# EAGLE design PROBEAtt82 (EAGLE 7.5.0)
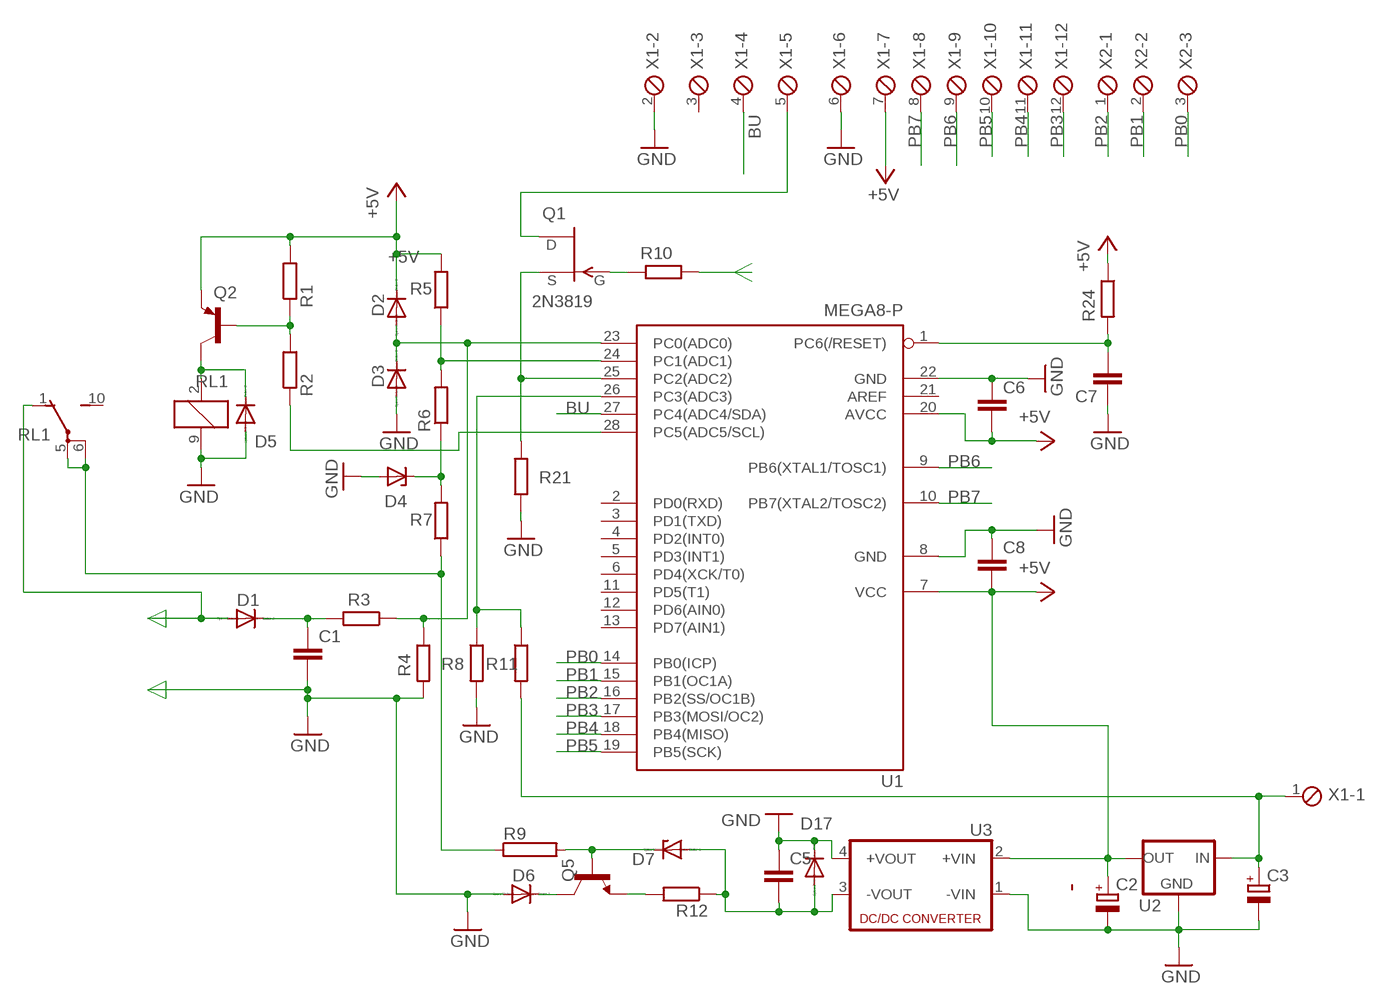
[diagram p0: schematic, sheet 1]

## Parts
C1  C-EU150-091X182  [C150-091X182]
C2  CPOL-EUE2-5  [E2-5]
C3  CPOL-EUE2-5  [E2-5]
C5  C-EUC1206  [C1206]
C6  C-EUC1206  [C1206]
C7  C-EUC1206  [C1206]
C8  C-EUC1206  [C1206]
D1  1N4004  [DO41-10]
D2  1N4004  [DO41-10]
D3  1N4004  [DO41-10]
D4  ZY  [P1Z12]
D5  1N4004  [DO41-10]
D6  1N4004  [DO41-10]
D7  DIODE-DO214AA  [DO214AA]
D17  DIODE-DO214AA  [DO214AA]
Q1  2N3819  [TO92]
Q2  BC327  [TO92]
Q5  -NPN-TO126  [TO126]
R1  R-EU_0204/7  [0204/7]
R2  R-EU_0204/7  [0204/7]
R3  R-EU_0617/22  [0617/22]
R4  R-EU_0411/12  [0411/12]
R5  R-EU_0204/7  [0204/7]
R6  R-EU_0204/7  [0204/7]
R7  R-EU_0414/15  [0414/15]
R8  R-EU_0204/7  [0204/7]
R9  RHPS932  [HPS932]
R10  R-EU_0204/7  [0204/7]
R11  R-EU_0204/7  [0204/7]
R12  R-EU_0204/7  [0204/7]
R21  R-EU_0204/7  [0204/7]
R24  R-EU_0204/7  [0204/7]
RL1  G5V1  [G5V1]
U1  MEGA8-P  [DIL28-3]
U2  78XXL  [78XXL]
U3  NME  [NME]
X1  MPT12  [12POL254]
X2  MPT3  [3POL254]

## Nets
+5V: C2.+ C6.2 C8.2 D2.C Q2.1(E) R1.2 R5.2 R24.1 U1.7(VCC) U1.20(AVCC) U2.OUT U3.2(+VIN) X1.7
BU: U1.27(PC4(ADC4/SDA)) X1.4
GND: C1.2 C2.- C3.- C5.1 C6.1 C7.1 C8.1 D3.A D4.A D5.A D6.A D17.C R4.2 R8.2 R21.2 RL1.9 U1.8(GND) U1.22(GND) U2.GND U3.1(-VIN) U3.4(+VOUT) X1.2 X1.6
N$1: R8.1 R11.1 U1.26(PC3(ADC3))
N$2: Q1.1(D) X1.5
N$3: C7.2 R24.2 U1.1(PC6(/RESET))
N$5: R5.1 R6.2 U1.24(PC1(ADC1))
N$6: D7.C Q5.3(B) R9.2
N$7: D4.C R6.1 R7.2
N$8: C1.1 D1.C R3.2
N$10: R2.1 U1.28(PC5(ADC5/SCL))
N$12: D5.C Q2.3(C) RL1.2
N$13: Q1.3(S) R21.1 U1.25(PC2(ADC2))
N$15: Q2.2(B) R1.1 R2.2
N$16: R7.1 R9.1 RL1.5(2:P) RL1.6(2:P)
N$18: C3.+ R11.2 U2.IN X1.1
N$19: D2.A D3.C R3.1 R4.1 U1.23(PC0(ADC0))
N$21: Q1.2(G) R10.2
N$28: C5.2 D7.A D17.A R12.1 U3.3(-VOUT)
N$30: Q5.1(E) R12.2
N$31: D6.C Q5.2(C)
N$32: R10.1
N$33: D1.A RL1.1(2:O)
PB0: U1.14(PB0(ICP)) X2.3
PB1: U1.15(PB1(OC1A)) X2.2
PB2: U1.16(PB2(SS/OC1B)) X2.1
PB3: U1.17(PB3(MOSI/OC2)) X1.12
PB4: U1.18(PB4(MISO)) X1.11
PB5: U1.19(PB5(SCK)) X1.10
PB6: U1.9(PB6(XTAL1/TOSC1)) X1.9
PB7: U1.10(PB7(XTAL2/TOSC2)) X1.8
Unconnected: RL1.10(2:S) U1.2(PD0(RXD)) U1.3(PD1(TXD)) U1.4(PD2(INT0)) U1.5(PD3(INT1)) U1.6(PD4(XCK/T0)) U1.11(PD5(T1)) U1.12(PD6(AIN0)) U1.13(PD7(AIN1)) U1.21(AREF) X1.3

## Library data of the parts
C1 C5-C8 = rcl:C-EU: CAPACITOR, European symbol
C2 C3 = rcl:CPOL-EU: POLARIZED CAPACITOR, European symbol
D1-D3 D5 D6 = diode:1N4004: DIODE
D4 = diode:ZY: Z DIODE
D7 D17 = diode:DIODE-: DIODE
Q1 = transistor-fet:2N3819: N-Channel Junction FET
Q2 = transistor-pnp:BC327: PNP Transistor
Q5 = transistor:*-NPN-: NPN Transistror BF959 corrected 2008.03.06
R1-R8 R10-R12 R21 R24 = rcl:R-EU_: RESISTOR, European symbol
R9 = resistor-power:R: Power Resitor; OC_FARNELL: unknown; OC_NEWARK: unknown
RL1 = relay:G5V1: RELAY 1 x switch, 0.5 A/125 V AC, 1 A/24 V DC , Omron; MPN: G5V-1-DC24; OC_FARNELL: 9949593; OC_NEWARK: 36M6377
U1 = atmel:MEGA8-P: MICROCONTROLLER 8 Kbytes FLASH, 1 kbytes SRAM, 512 bytes EEPROM, USART, 4-channel 10 bit ADC, 2-channel 8 bit ADC Pin compatible with Atmega48, ATMega88, ATMega168 Source: avr.lbr; OC_FARNELL: unknown; OC_NEWARK: unknown
U2 = v-reg:78XXL: VOLTAGE REGULATOR
U3 = dc-dc-converter:NME: DC-DC CONVERTER; MF: C & D TECHNOLOGIES, INC; MPN: NME1205D; OC_FARNELL: 1021466; OC_NEWARK: 98B8198
X1 = con-phoenix-254:MPT12: PHOENIX CONNECTOR; OC_FARNELL: unknown; OC_NEWARK: unknown
X2 = con-phoenix-254:MPT3: PHOENIX CONNECTOR; OC_FARNELL: unknown; OC_NEWARK: unknown

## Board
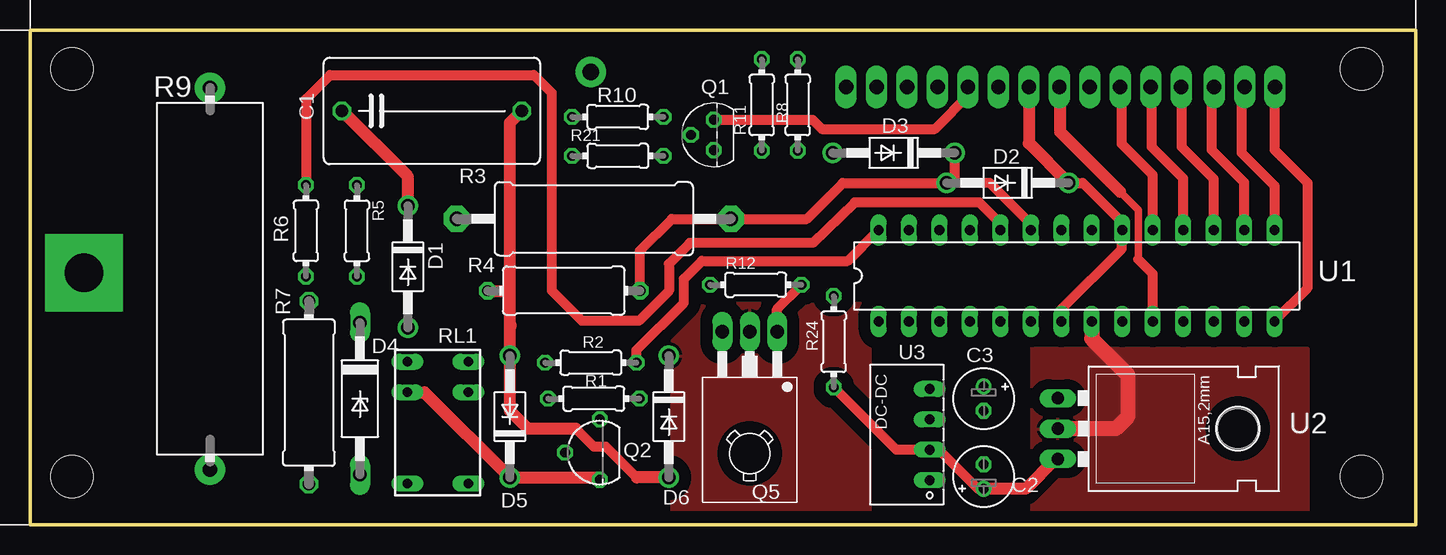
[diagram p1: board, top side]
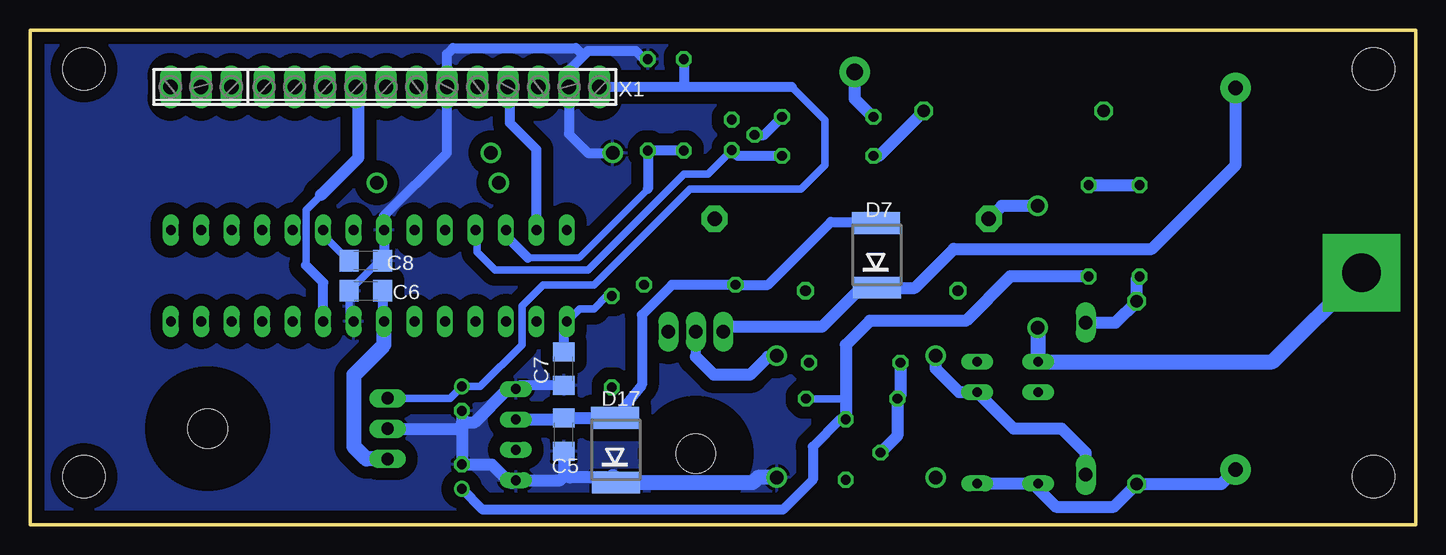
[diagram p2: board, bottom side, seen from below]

Size 115.5 x 41.25 mm. Coordinates in mm from the lower left corner, seen from the top.
Outline: 0,0 0,41.25 115.5,41.25 115.5,0 0,0
Copper layers (1*16): Top 0.035mm / dielectric 1.5mm / Bottom 0.035mm
Design rules "default": minimum track width 10mil, minimum drill 24mil, track to track 8mil, track to pad 8mil, pad to pad 8mil, via to via 8mil, smd to smd 8mil, copper to edge 40mil, drill to drill 8mil, minimum pad ring 10mil, minimum via ring 8mil, stop-mask expansion 4mil, vias tented up to drill 0mil, thermal gap 10mil
Holes 3.5 mm at 3.5,38 3.5,4 111,4 111,38

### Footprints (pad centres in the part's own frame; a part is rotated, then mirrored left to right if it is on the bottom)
C150-091X182 = drill 1.016 octagon: 1 -7.493,0; 2 7.493,0
E2-5 = drill 0.813 pad 1.27: + -1.016,0 | drill 0.813 pad 1.27 octagon: - 1.016,0
C1206 = smd 1.6 x 1.8: 1 -1.4,0; 2 1.4,0
DO41-10 = drill 1.118: A 5.08,0; C -5.08,0
P1Z12 = drill 1.118 long: A 6.35,0; C -6.35,0
DO214AA = smd 1.8 x 4: A 2.65,0; C -2.75,-0.1
TO92 = drill 0.813 octagon: 1 1.27,0; 2 0,1.905; 3 -1.27,0
TO92' = drill 0.813 octagon: 1 2.77,0; 2 0,2.905; 3 -2.27,0
TO126 = drill 1.118 long: 1 -2.286,-5.08; 2 0,-5.08; 3 2.286,-5.08 | hole 3.302: 0,5.08
0204/7 = drill 0.813 octagon: 1 -3.81,0; 2 3.81,0
0617/22 = drill 1.2 pad 2.184 octagon: 1 -11.43,0; 2 11.43,0
0411/12 = drill 0.914 octagon: 1 -6.35,0; 2 6.35,0
0414/15 = drill 1.016 octagon: 1 -7.62,0; 2 7.62,0
HPS932 = drill 1.2 pad 2.54: 1 -15.93,0; 2 15.93,0
G5V1 = drill 0.813 long: 1 -5.08,-2.54; 2 -2.54,-2.54; 5 5.08,-2.54; 6 5.08,2.54; 9 -2.54,2.54; 10 -5.08,2.54
DIL28-3 = drill 0.813 long: 1 -16.51,-3.81; 2 -13.97,-3.81; 3 -11.43,-3.81; 4 -8.89,-3.81; 5 -6.35,-3.81; 6 -3.81,-3.81; 7 -1.27,-3.81; 8 1.27,-3.81; 9 3.81,-3.81; 10 6.35,-3.81; 11 8.89,-3.81; 12 11.43,-3.81; 13 13.97,-3.81; 14 16.51,-3.81; 15 16.51,3.81; 16 13.97,3.81; 17 11.43,3.81; 18 8.89,3.81; 19 6.35,3.81; 20 3.81,3.81; 21 1.27,3.81; 22 -1.27,3.81; 23 -3.81,3.81; 24 -6.35,3.81; 25 -8.89,3.81; 26 -11.43,3.81; 27 -13.97,3.81; 28 -16.51,3.81
78XXL = drill 1.016 long: GND 0,-3.81; IN -2.54,-3.81; OUT 2.54,-3.81 | hole 3.302: 0,11.176
NME = drill 0.813 long: 1 0,3.81; 2 0,1.27; 3 0,-1.27; 4 0,-3.81
12POL254 = drill 1.2 long: 1 -13.97,0; 2 -11.43,0; 3 -8.89,0; 4 -6.35,0; 5 -3.81,0; 6 -1.27,0; 7 1.27,0; 8 3.81,0; 9 6.35,0; 10 8.89,0; 11 11.43,0; 12 13.97,0
3POL254 = drill 1.2 long: 1 -2.54,0; 2 0,0; 3 2.54,0

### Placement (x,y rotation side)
C1  33.5,34.5 0 top
C2  79.5,4 90 top
C3  79.5,10.5 270 top
C5  71,7.5 90 bottom
C6  87.5,19.5 0 bottom
C7  71,13 90 bottom
C8  87.5,22 180 bottom
D1  31.5,21.5 270 top
D2  81.5,28.5 180 top
D3  72,31 180 top
D4  27.5,10.5 270 top
D5  40,9 90 top
D6  53.25,9 270 top
D7  45,22.5 90 bottom
D17  66.75,6.25 90 bottom
Q1  57,32.5 90 top
Q2  BC327  [TO92']  47.5,6 90 top
Q5  60,11 180 top
R1  47,10.5 0 top
R2  46.75,13.5 180 top
R3  47,25.5 180 top
R4  44.5,19.5 180 top
R5  27.25,24.5 270 top
R6  23,24.5 90 top
R7  23.25,11 90 top
R8  64,35 90 top
R9  15,20.5 90 top
R10  49,34 0 top
R11  61,35 90 top
R12  60.5,20 0 top
R21  49,30.75 180 top
R24  67,15.25 90 top
RL1  34,8.5 270 top
U1  87.25,20.75 0 top
U2  89.5,8 270 top
U3  75,7.5 180 top
X1  82,36.5 180 bottom
X2  101.25,36.5 180 bottom

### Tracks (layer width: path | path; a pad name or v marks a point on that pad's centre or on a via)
+5V
  Top 0.813: C2.+ 79.48,3 79,3 75.77,6.23 U3.2 72.21,6.23 R24.1 | U1.7 85.98,17.98 91,23 91,24.5 U1.20 91,24.62 91,25.25 87.75,28.5 87.12,28.5
  Top 1.016: U2.OUT 85.46,5.46 83,3 79.52,3 C2.+ | X1.7 83.27,31.81 D2.C 87.12,28.5
  Bottom 0.61: U1.20 91.06,24.16 C8.2 | R1.2 47.5,10.5
  Bottom 0.813: C6.2 86.1,17.06 U1.7 | Q2.1 47.98,8.77 50.25,6.5 50.25,3.75 52.75,1.25 77.77,1.25 C2.+
  Bottom 1.016: R5.2 33.81,20.69 37.5,17 45.5,17 47.5,15 47.5,10.5 Q2.1
  Bottom 1.27: U2.OUT 87.46,5.46 88.5,6.5 88.5,12.5 86,15 86,16.92 U1.7
BU
  Bottom 0.813: U1.27 73.28,31.28 75.5,33.5 75.5,35.85 X1.4
GND
  Top 0.813: 50.58,3.92 48,6.5 47,6.5 45.5,8
  Top 1.016: 40,16.5 D5.A 40,9.5 41.5,8 45.5,8 | 40,16.5 40,19.5 | 40,19.5 40,33.51 C1.2 | R4.2 40,19.5 | 40.08,16.58 40,16.5 | D6.A 50.58,3.92
  Top 1.27: U1.8 88.52,15.48 91.5,12.5 91.5,9 90.5,8 U2.GND
  Bottom 0.61: C8.1 86.4,22 C6.1 88.9,17.32 U1.8
  Bottom 0.813: C7.1 74.71,11.6 U3.4 | R8.2 64.31,38.81 65,39.5 69,39.5 69.38,39.12 | 69.38,39.12 70.5,38 70.5,36.57 X1.2 70.57,32.57 69,31 D3.A | C8.1 85.98,22.12 U1.22 85.98,25.77 80.75,31 80.75,36.48 X1.6 80.73,39.23 80.75,39.25 80.25,39.75 70,39.75 69.38,39.12
  Bottom 1.016: R21.2 44.74,30.75 C1.2 | D5.A 40,13 38.04,11.04 RL1.9 33.5,8 29.5,8 27.5,6 D4.A | C5.1 71,4.42 70.79,4.21 | 70.79,4.21 70.5,3.92 67,3.92 66.9,4.02 D17.C | 70.79,4.21 71.31,3.69 U3.1 75.19,3.5 75.5,3.5 77.02,5.02 C2.- 79.5,8 | C3.- 79.5,8.5 | 79.5,8.5 79.5,8 | U2.GND 79.5,8 | U3.4 75.69,11.31 78.5,8.5 79.5,8.5
  Bottom 1.27: D6.A 54.83,3.92 55.25,3.5 66.38,3.5 66.9,4.02
  pour Bottom (isolate 1.016): 50.5,40.5 114.75,40.5 114.75,0.75 50.5,0.75
  pour Top (isolate 0.813): 106.5,14.75 106.5,1 83.5,1 83.5,14.75
N$1
  Bottom 0.6: 64,28 69.75,22.25 74,22.25
  Bottom 0.813: R11.1 R8.1 64,28 | 74,22.25 75.75,24 75.75,24.49 U1.26
N$2
  Top 0.813: Q1.1 65.23,33.77 66,33 75.44,33 78.4,35.96 | 78.5,35.69 78.4,35.96 | 78.4,35.96 X1.5
N$3
  Bottom 0.61: R24.2 67.44,19.06 68.5,18 69.68,18 U1.1
  Bottom 0.813: C7.2 71,16.68 U1.1
N$4  (via drill 1.4 pad 2.54)
  Bottom 1.016: 45.25,34 46.75,35.5 v46.75,37.75 47,37.75
N$5
  Top 0.813: U1.24 80.9,25.1 79.12,26.88 68.75,26.88 65.25,23.5 55,23.5 53.25,21.75 53.25,19.5 50.75,17 46,17 43.5,19.5 43.5,36 42,37.5 25,37.5 23,35.5 R6.2
  Bottom 1.016: R5.1 R6.2
N$6
  Bottom 1.016: R9.2 15,30 22,23 38.5,23 41.75,19.75 D7.C 46.25,19.75 49.5,16.5 57.29,16.5 Q5.3
N$7
  Bottom 1.016: R6.1 23.25,20.44 R7.2 25.02,16.85 D4.C
N$8
  Top 1.016: D1.C 31.5,29.01 C1.1
  Bottom 1.016: D1.C 34.49,26.58 R3.2
N$10
  Top 0.813: R2.1 50.56,14.56 54.5,18.5 54.5,20.5 56,22 68.18,22 U1.28
N$12
  Top 1.016: RL1.2 32.88,11.04 D5.C 47.31,3.92 Q2.3
N$13
  Bottom 0.61: U1.25 78.25,24.45 78.25,22.75 76.75,21.25 69,21.25 61,29.25 58.98,29.25 Q1.3
  Bottom 0.813: R21.1 56.52,30.75 Q1.3 57.02,31.23
N$15
  Bottom 1.016: R2.2 42.94,10.75 R1.1 43.19,7.41 Q2.2
N$16
  Bottom 1.016: RL1.6 RL1.5 31.46,2.96 30,1.5 25.13,1.5 R7.1 16.19,3.38 R9.1
N$18
  Bottom 0.61: U2.IN 80.48,10.54 C3.+ 77.98,11.52 74.5,15 74.5,18.25 72.75,20 68.5,20 60.5,28 51.25,28 49.25,30 49.25,33.75 52,36.5
  Bottom 0.813: 52,36.5 61,36.5 | 61,36.5 X1.1 | R11.2 61,36.5
N$19
  Top 0.813: R4.1 50.85,22.85 53.5,25.5 R3.1 64.75,25.5 67.75,28.5 D2.A 77,28.5 | U1.23 83.44,25.06 80,28.5 77,28.5 | D3.C 77.08,28.58 77,28.5
N$21
  Bottom 0.813: Q1.2 54.31,32.5 R10.2
N$28
  Bottom 0.813: D17.A 64.5,11.65 64.5,17.5 62,20 R12.1 54,20 48.75,25.25 45.1,25.25 D7.A
  Bottom 1.016: U3.3 71.13,8.77 C5.2 D17.A
N$30
  Top 0.813: Q5.1 62.29,17.98 R12.2
N$31
  Bottom 0.813: 60,14 Q5.2
  Bottom 1.016: D6.C 54,14 55.5,12.5 58.5,12.5 60,14
  pour Top (isolate 1.016): 55.75,18.5 70,18.5 70,0.5 53.5,0.5 53.5,16.25
N$33  (via drill 3.2 pad 6.45)
  Bottom 1.27: v4.5,21 11.92,13.58 RL1.1 31.5,13.62 D1.A
PB0
  Top 0.813: U1.14 103.76,17.01 106.5,19.75 106.5,28.5 103.75,31.25 103.75,36.46 X2.3
PB1
  Top 0.813: U1.15 103.76,28.24 101,31 101,36.25 X2.2
PB2
  Top 0.813: U1.16 101.22,28.53 98.5,31.25 98.5,36.29 X2.1
PB3
  Top 0.813: U1.17 98.68,28.82 96,31.5 96,36.47 X1.12
PB4
  Top 0.813: U1.18 96.14,28.86 93.5,31.5 93.5,36.43 X1.11
PB5
  Top 0.813: U1.19 93.6,29.15 91,31.75 91,36.39 X1.10
PB6
  Bottom 0.61: 92.5,21.62 92.5,26.25 91.25,27.5
  Bottom 0.813: U1.9 91.06,20.18 92.5,21.62
  Bottom 1.016: 91.25,27.5 88.12,30.62 88.12,36.27 X1.9
PB7
  Top 0.61: 92.38,22.12 92.38,26.25 90.88,27.75
  Top 0.813: U1.10 93.6,20.9 92.38,22.12
  Top 1.016: 90.88,27.75 85.88,32.75 85.88,36.44 X1.8

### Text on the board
tNames: R1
